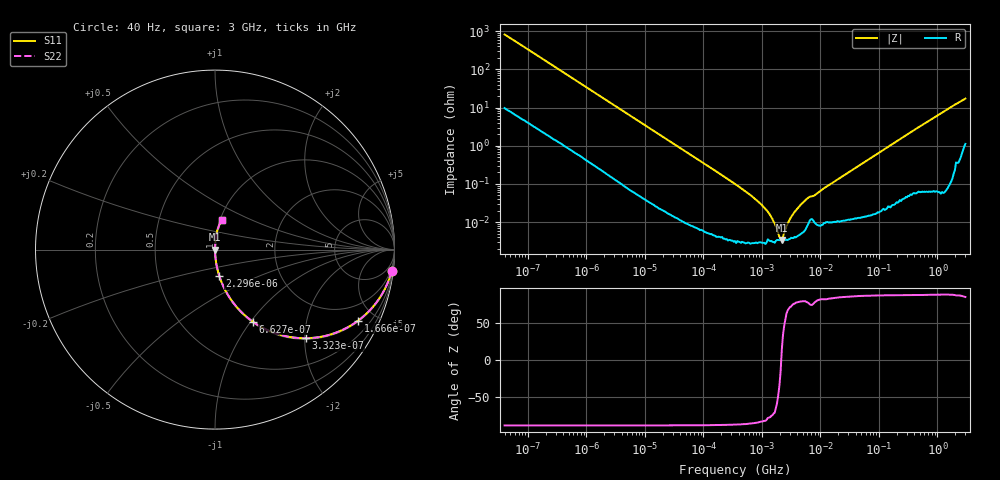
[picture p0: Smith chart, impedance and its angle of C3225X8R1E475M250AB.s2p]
! S-parameter Generated by TDK Corporation
! Copyright(C) 2015 TDK Corporation.
! All Rights Reserved.
! TDK P/N: C3225X8R1E475M250AB (Multilayer Ceramic Chip Capacitors)
! Property: C=4.7uF
! Size(LxWxT): 3.2x2.5x2.5mm, 0.126x0.098x0.098inches
! Model Type: s2p (Touchstone File Format Version 1.0)
! Frequency: DC=Yes Start=0.00004MHz Stop=3000MHz 396points Log-sweep
! Note: This model was converted from impedance.
! Model Generated on Jun. 23, 2015
! Hash(MD5):
! Port Assignments:
!  1 ---| |--- 2
! Applicable Conditions:
!  Temperature = 25 degC
!  DC Bias Voltage = 0 V
!  Small Signal Operation
! Terms and conditions regarding TDK Simulation Models
! (1)This simulation model is being provided solely for informational purposes. Please refer to the specifications of the products in terms of detailed characteristics of such products.
! (2)In no event shall TDK Corporation of any of its subsidiaries be liable for any loss or damage arising, directly or indirectly,
!  From any information contained in this simulation model, including, but not limited to loss or damages arising from any inaccuracies, omissions or errors in connection with such information.
! (3)Any and all copyrights on this simulation model are owned by TDK Corporation.
!  Duplication or redistribution of this simulation model without prior written permission from TDK Corporation is prohibited.
! (4)This simulation model is subject to any modification or change without any prior notice.
! (5)Neither TDK Corporation nor any of its subsidiaries shall make any warranty, express or implied,
!  Including but not limited to the correctness, implied warranties of merchantability and fitness for a particular purpose with respect to this simulation models.
! (6)The use of this simulation model shall be deemed to have consented to the terms and conditions hereof.
# MHz S MA R 50
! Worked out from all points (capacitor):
!   395 points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, 40 Hz to 3 GHz, reference 50 ohm
!   read as one part in series: C = 4.84 uF near 41.88 Hz
!   lowest |Z| = 3.45 mohm at 2.183 MHz (marker M1)
!   series resonance near 2.138 MHz, so ESL is about 1.1 nH
!   S11 on the Smith chart (normalised r, x): 40 Hz: 1, -16; 166.6 Hz: 1.05, -4.01; 332.3 Hz: 1.02, -2.03; 662.7 Hz: 1.01, -1.02; 2.296 kHz: 1.00, -0.30; 3 GHz: 1.02, +0.34
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4e-05  0.9912 -7.0  0.1214 82.3  0.1214 82.3  0.9912 -7.0
9.158711e-05  0.9611 -15.4  0.2648 74.0  0.2648 74.0  0.9611 -15.4
0.0001665986  0.8908 -26.3  0.4437 63.0  0.4437 63.0  0.8908 -26.3
0.0003322641  0.7072 -44.3  0.6984 45.0  0.6984 45.0  0.7072 -44.3
0.000662667  0.4529 -62.4  0.8861 26.9  0.8861 26.9  0.4529 -62.4
0.000834128  0.3753 -67.2  0.9223 22.0  0.9223 22.0  0.3753 -67.2
0.002295921  0.1476 -80.8  0.9873 8.5  0.9873 8.5  0.1476 -80.8
0.005504511  0.06272 -85.8  0.9973 3.6  0.9973 3.6  0.06272 -85.8
0.01739424  0.02007 -88.2  0.9996 1.2  0.9996 1.2  0.02007 -88.2
0.3464102  0.001003 -88.1  1 0.1  1 0.1  0.001003 -88.1
0.9534872  0.000301 -84.3  1 0.0  1 0.0  0.000301 -84.3
1.256723  0.0001893 -79.2  1 0.0  1 0.0  0.0001893 -79.2
1.581893  0.0001035 -73.1  1 0.0  1 0.0  0.0001035 -73.1
2.183178  3.452e-05 13.5  1 -0.0  1 -0.0  3.452e-05 13.5
2.877491  0.0001059 70.4  1 -0.0  1 -0.0  0.0001059 70.4
3.622024  0.0001866 77.2  1 -0.0  1 -0.0  0.0001866 77.2
4.5592  0.0002825 80.1  1 -0.0  1 -0.0  0.0002825 80.1
6.009156  0.0004223 78.7  0.9999 -0.0  0.9999 -0.0  0.0004223 78.7
7.22376  0.0004774 75.5  0.9999 -0.0  0.9999 -0.0  0.0004774 75.5
150.6385  0.009928 88.0  0.9997 -0.6  0.9997 -0.6  0.009928 88.0
865.884  0.05427 86.2  0.9979 -3.1  0.9979 -3.1  0.05427 86.2
3000  0.167 76.6  0.9751 -9.6  0.9751 -9.6  0.167 76.6
